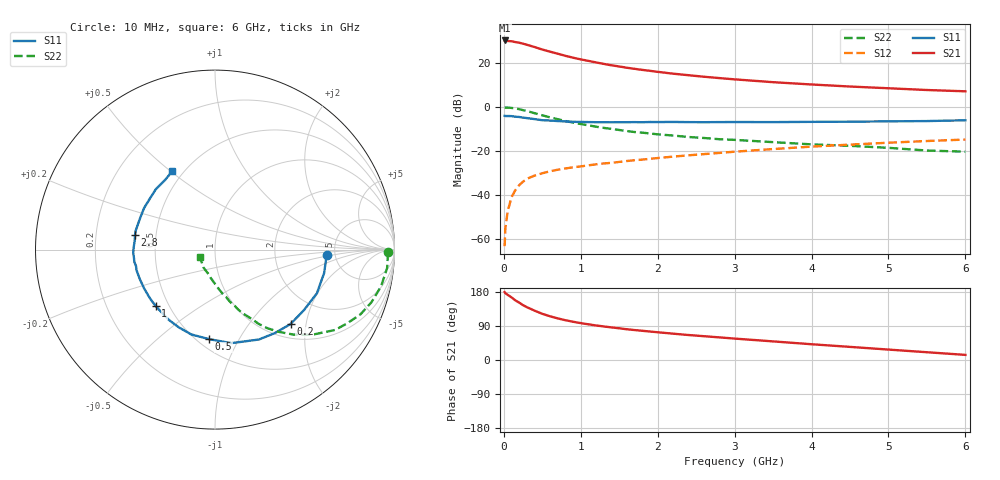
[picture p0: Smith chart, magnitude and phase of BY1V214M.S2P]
! SIEMENS Small Signal Semiconductors
! BFY420
! Si NPN RF SIEGET Grounded Emitter Transistor in MICRO-X
! VCE = 1.25 V  IC = 14 mA
! Common Emitter S-Parameters:  October  1996
# GHz  S  MA  R  50
!  f  S11  S21  S12  S22
! GHz  MAG  ANG  MAG  ANG  MAG  ANG  MAG  ANG
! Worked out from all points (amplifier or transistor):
!   36 points, 10 MHz to 6 GHz, reference 50 ohm
!   highest |S21| = 30.1 dB at 10 MHz (marker M1)
!   |S21| within 3 dB of that: start of sweep to 401.3 MHz
!   unconditionally stable (mu >= 1): 2.163 GHz to end of sweep
!   at 250 MHz: K = 0.25, MSG = 31.2 dB, |S12| = -33.9 dB
!   at 1.4 GHz: K = 0.85, MSG = 22.1 dB, |S12| = -25.4 dB
!   at 6 GHz: K = 1.10, MAG = 9.0 dB, |S12| = -14.8 dB
!   S11 on the Smith chart (normalised r, x): 10 MHz: 4.29, -0.40; 200 MHz: 1.28, -1.63; 500 MHz: 0.57, -0.76; 1 GHz: 0.42, -0.34; 2.8 GHz: 0.38, +0.08; 6 GHz: 0.44, +0.51
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0.01  0.6246 -2.6  31.99 179.1  0.0007 102.5  0.9646 -0.9
0.02  0.6212 -5.0  31.79 176.2  0.0018 94.2  0.9635 -2.2
0.1  0.6178 -23.2  30.66 165.2  0.009 82.8  0.9476 -12.5
0.15  0.5994 -34.2  29.45 157.2  0.0131 74.4  0.9197 -18.6
0.2  0.591 -44.6  28.39 151.3  0.0169 72.0  0.887 -24.0
0.25  0.5717 -54.7  27.01 144.7  0.0203 66.6  0.8437 -29.1
0.3  0.5573 -64.0  25.55 139.3  0.0235 64.6  0.8049 -33.8
0.4  0.5292 -80.1  22.69 130.2  0.0278 59.7  0.7194 -41.3
0.5  0.5 -93.7  19.93 121.8  0.0314 56.1  0.6442 -47.3
0.6  0.4909 -105.5  17.84 115.4  0.0348 54.1  0.58 -52.2
0.7  0.478 -114.8  16.04 109.8  0.0377 52.9  0.5266 -56.3
0.8  0.4686 -123.2  14.36 105.0  0.0402 51.0  0.4791 -59.6
1  0.4562 -136.4  11.9 97.4  0.0449 50.5  0.409 -64.4
1.1  0.4531 -142.7  11.01 94.1  0.0474 50.7  0.3818 -67.0
1.4  0.4491 -155.4  8.737 86.0  0.054 50.6  0.3176 -72.4
1.6  0.4504 -162.4  7.706 81.1  0.0595 50.3  0.2833 -75.7
2.2  0.4561 -178.2  5.657 69.5  0.0748 49.2  0.2245 -83.9
2.8  0.4528 169.9  4.497 59.7  0.0906 46.7  0.1855 -91.2
3.5  0.4525 157.7  3.628 49.1  0.1109 43.2  0.1591 -98.8
4.5  0.4612 141.6  2.894 34.6  0.1398 35.5  0.1313 -111.1
5.5  0.4775 125.6  2.413 20.5  0.1688 26.4  0.1027 -135.7
6  0.4976 118.5  2.254 13.5  0.1821 21.8  0.0966 -153.0
